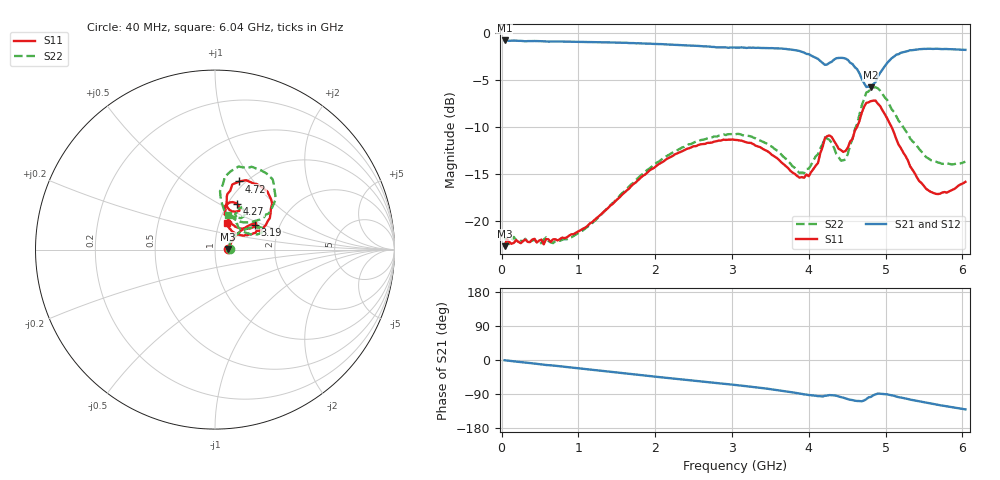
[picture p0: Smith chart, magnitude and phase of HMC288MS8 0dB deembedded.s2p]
!Hittite Microwave Corporation
!12 Elizabeth Drive
!Chelmsford, MA 01824
!Tel: 978-250-3343
!Fax: 978-250-3373
!Device: HMC288MS8, 0.7-3.7 GHz GaAs IC 3-bit Digital Attenuator in 8-lead Grounded Base surface Mount Plastic Package
!Misc:  0dB state, Room
# GHZ S DB R 50.0
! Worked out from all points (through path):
!   201 points, 40 MHz to 6.04 GHz, reference 50 ohm
!   highest |S21| = -0.84 dB at 40 MHz (marker M1); lowest = -5.8 dB at 4.81 GHz (marker M2)
!   group delay of S21, straight-line fit = 57 ps
!   lowest |S11| = -22.6 dB at 40 MHz (marker M3), VSWR 1.16, Z = 57.9 + j0.46 ohm
!   |S11| at or under -10 dB: start of sweep to 4.629 GHz; 5.079 GHz to end of sweep
!   |S22| runs from -22.4 to -5.8 dB; largest |S21 - S12| = 0.0057
!   S11 on the Smith chart (normalised r, x): 40 MHz: 1.16, +0.01; 3.19 GHz: 1.50, +0.44; 4.27 GHz: 1.10, +0.62; 4.72 GHz: 0.94, +0.85; 6.04 GHz: 1.09, +0.33
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0.04  -22.65 3.1  -0.84 -0.6  -0.87 -0.4  -21.75 3.1
0.67  -21.93 6.8  -0.95 -14.5  -0.95 -14.7  -22.32 7.0
1.06  -20.80 19.8  -0.99 -23.2  -0.99 -23.3  -20.97 22.6
2.05  -13.93 36.0  -1.22 -45.0  -1.22 -45.1  -13.67 33.6
3.04  -11.38 31.5  -1.59 -65.8  -1.58 -65.9  -10.81 22.6
3.19  -11.64 31.1  -1.63 -69.2  -1.60 -69.5  -10.93 20.9
3.52  -12.97 31.2  -1.65 -77.3  -1.63 -77.5  -12.10 19.8
3.88  -15.38 49.0  -1.96 -88.5  -1.94 -88.7  -14.88 36.7
4.06  -14.47 68.7  -2.56 -93.9  -2.56 -94.1  -13.58 57.6
4.18  -12.15 77.6  -3.21 -96.4  -3.17 -96.5  -11.86 61.5
4.27  -10.91 64.3  -3.21 -92.5  -3.21 -92.7  -11.38 50.5
4.42  -12.47 63.0  -2.68 -97.8  -2.66 -98.0  -13.58 59.8
4.48  -12.55 70.0  -2.76 -101.5  -2.75 -101.5  -13.45 71.6
4.63  -9.99 77.5  -3.88 -108.2  -3.88 -108.4  -9.70 85.1
4.72  -7.89 70.4  -5.34 -106.9  -5.36 -106.6  -7.05 78.8
4.81  -7.27 57.6  -5.78 -97.3  -5.77 -97.7  -5.94 66.2
4.9  -7.54 41.9  -4.66 -88.7  -4.64 -88.8  -5.91 50.7
5.05  -9.58 28.2  -2.97 -91.9  -2.94 -92.2  -7.63 38.0
5.2  -12.26 22.5  -2.14 -98.9  -2.15 -99.0  -9.66 33.5
5.53  -16.57 36.6  -1.73 -112.8  -1.72 -112.9  -13.22 43.8
5.8  -16.97 54.7  -1.75 -122.3  -1.75 -122.5  -13.87 58.9
6.04  -15.83 65.7  -1.84 -130.3  -1.82 -130.5  -13.69 69.4
